(* Logix 5000 AddOnInstructionDefinition export Valve_Disc; software revision 20.01 *)

TYPE Valve_Disc_Type :   // Discrete Valve data
STRUCT
   Open_Status : BOOL;   // Open LS status (1=open valve)
   Close_Status : BOOL;   // Close LS status (1=closed valve)
   Any_Fail : BOOL;   // Overall Failure Alarm (1= alarm)
   FTO_Fail : BOOL;   // Fail-to-open alarm (1=alarm)
   FTC_Fail : BOOL;   // Fail-to-close alarm (1=alarm)
   Seq_Open : BOOL;   // Valve open initiated from sequence
   Seq_Close : BOOL;   // Valve close initiated from sequence
END_STRUCT
END_TYPE

ADD_ON_INSTRUCTION Valve_Disc   (* revision 1.5 *)
// Discrete Valve Control
// Revision note:
// Correct name of "Dev_Num" input parameters
VAR_INPUT
   Open_LS : BOOL; {required}   // Valve-Open limit switch
   Close_LS : BOOL; {required}   // Valve-Closed limit switch
   Alarm_Reset : BOOL; {required}   // Resets alarms
   Maint : BOOL; {required}   // Unit Maintenance/Operate Privilege
   Man_Open : BOOL; {required}   // Manual start/open for unit
   Man_Close : BOOL; {required}   // Manual stop/close for unit
   Select_Dev_Num : DINT; {required}   // Number of device started/stopped at OI
   This_Dev_Num : DINT; {required}   // Number of this device for OI control
END_VAR
VAR_OUTPUT
   Vlv_Sol : BOOL; {access Read Only, required}   // Valve solenoid (1=open, 0=close)
END_VAR
VAR_IN_OUT
   Tag : Valve_Disc_Type; {required}   // Valve Tag
END_VAR
VAR
   Fail_Tmr : TIMER := (PRE := 20000);   // Timer for alarms
END_VAR

ROUTINE Logic   (* ladder *)
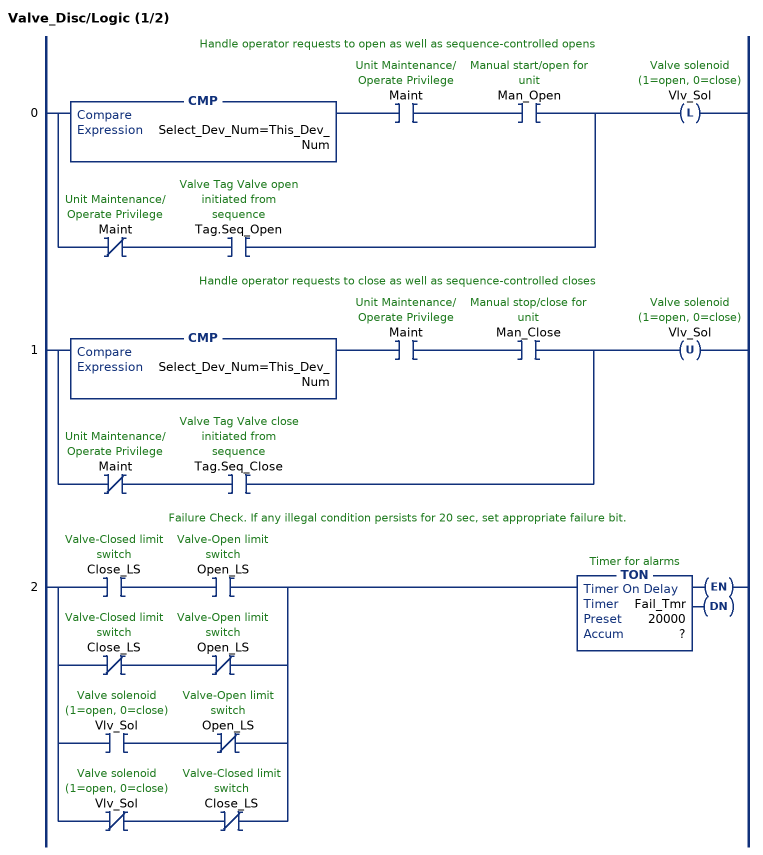
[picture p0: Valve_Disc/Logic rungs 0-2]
   // Handle operator requests to open as well as sequence-controlled opens
   0: [CMP(Select_Dev_Num=This_Dev_Num) XIC(Maint) XIC(Man_Open) ,XIO(Maint) XIC(Tag.Seq_Open) ]OTL(Vlv_Sol);
   // Handle operator requests to close as well as sequence-controlled closes
   1: [CMP(Select_Dev_Num=This_Dev_Num) XIC(Maint) XIC(Man_Close) ,XIO(Maint) XIC(Tag.Seq_Close) ]OTU(Vlv_Sol);
   // Failure Check. If any illegal condition persists for 20 sec, set appropriate failure bit.
   2: [XIC(Close_LS) XIC(Open_LS) ,XIO(Close_LS) XIO(Open_LS) ,XIC(Vlv_Sol) XIO(Open_LS) ,XIO(Vlv_Sol) XIO(Close_LS) ]TON(Fail_Tmr,?,?);
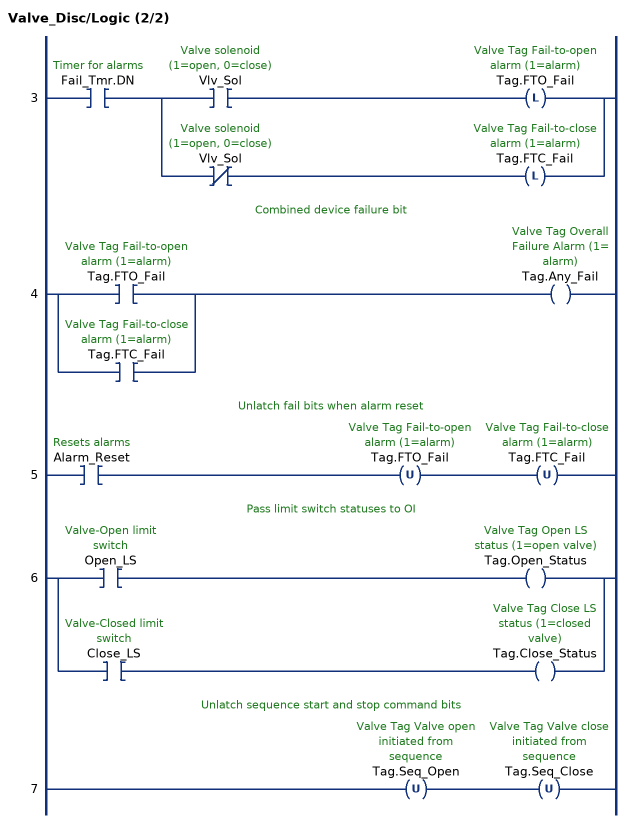
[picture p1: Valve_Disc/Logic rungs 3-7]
   3: XIC(Fail_Tmr.DN)[XIC(Vlv_Sol) OTL(Tag.FTO_Fail) ,XIO(Vlv_Sol) OTL(Tag.FTC_Fail) ];
   // Combined device failure bit
   4: [XIC(Tag.FTO_Fail) ,XIC(Tag.FTC_Fail) ]OTE(Tag.Any_Fail);
   // Unlatch fail bits when alarm reset
   5: XIC(Alarm_Reset)OTU(Tag.FTO_Fail)OTU(Tag.FTC_Fail);
   // Pass limit switch statuses to OI
   6: [XIC(Open_LS) OTE(Tag.Open_Status) ,XIC(Close_LS) OTE(Tag.Close_Status) ];
   // Unlatch sequence start and stop command bits
   7: OTU(Tag.Seq_Open)OTU(Tag.Seq_Close);
END_ROUTINE
END_ADD_ON_INSTRUCTION
